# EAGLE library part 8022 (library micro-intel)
MICROCOMPUTER/PERIPHERAL DEVICE
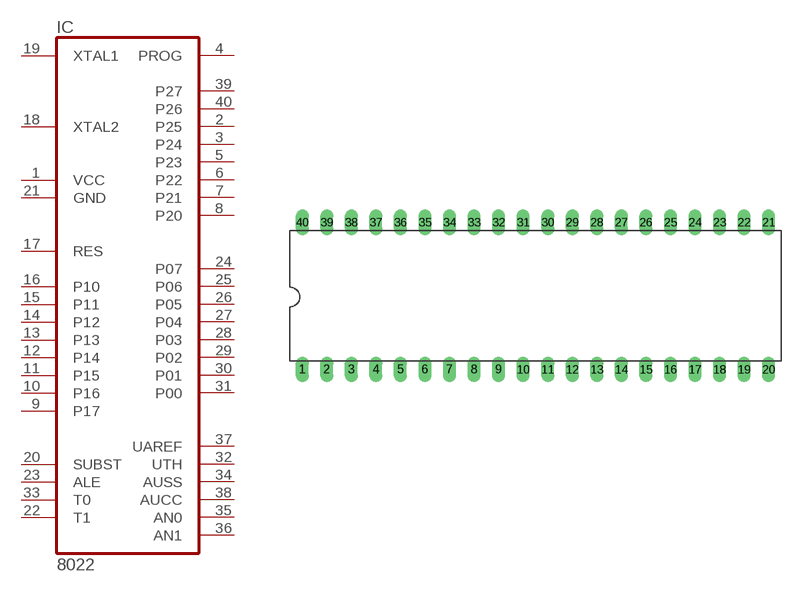
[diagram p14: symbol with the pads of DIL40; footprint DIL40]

Designator prefix IC

## 8022 (OC_FARNELL: unknown; OC_NEWARK: unknown)  [DIL40]
1  VCC  pwr
2  P25
3  P24
4  PROG  out
5  P23
6  P22
7  P21
8  P20
9  P17
10  P16
11  P15
12  P14
13  P13
14  P12
15  P11
16  P10
17  RES  in
18  XTAL2  in
19  XTAL1  in
20  SUBST  in
21  GND  pwr
22  T1  in
23  ALE  out
24  P07
25  P06
26  P05
27  P04
28  P03
29  P02
30  P01
31  P00
32  UTH  pwr
33  T0
34  AUSS  pwr
35  AN0  in
36  AN1  in
37  UAREF  pwr
38  AUCC  pwr
39  P27
40  P26

## Footprint DIL40 (pad centres in mm)
Dual In Line Package
drill 0.813 long: 1 -24.13,-7.62; 2 -21.59,-7.62; 3 -19.05,-7.62; 4 -16.51,-7.62; 5 -13.97,-7.62; 6 -11.43,-7.62; 7 -8.89,-7.62; 8 -6.35,-7.62; 9 -3.81,-7.62; 10 -1.27,-7.62; 11 1.27,-7.62; 12 3.81,-7.62; 13 6.35,-7.62; 14 8.89,-7.62; 15 11.43,-7.62; 16 13.97,-7.62; 17 16.51,-7.62; 18 19.05,-7.62; 19 21.59,-7.62; 20 24.13,-7.62; 21 24.13,7.62; 22 21.59,7.62; 23 19.05,7.62; 24 16.51,7.62; 25 13.97,7.62; 26 11.43,7.62; 27 8.89,7.62; 28 6.35,7.62; 29 3.81,7.62; 30 1.27,7.62; 31 -1.27,7.62; 32 -3.81,7.62; 33 -6.35,7.62; 34 -8.89,7.62; 35 -11.43,7.62; 36 -13.97,7.62; 37 -16.51,7.62; 38 -19.05,7.62; 39 -21.59,7.62; 40 -24.13,7.62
